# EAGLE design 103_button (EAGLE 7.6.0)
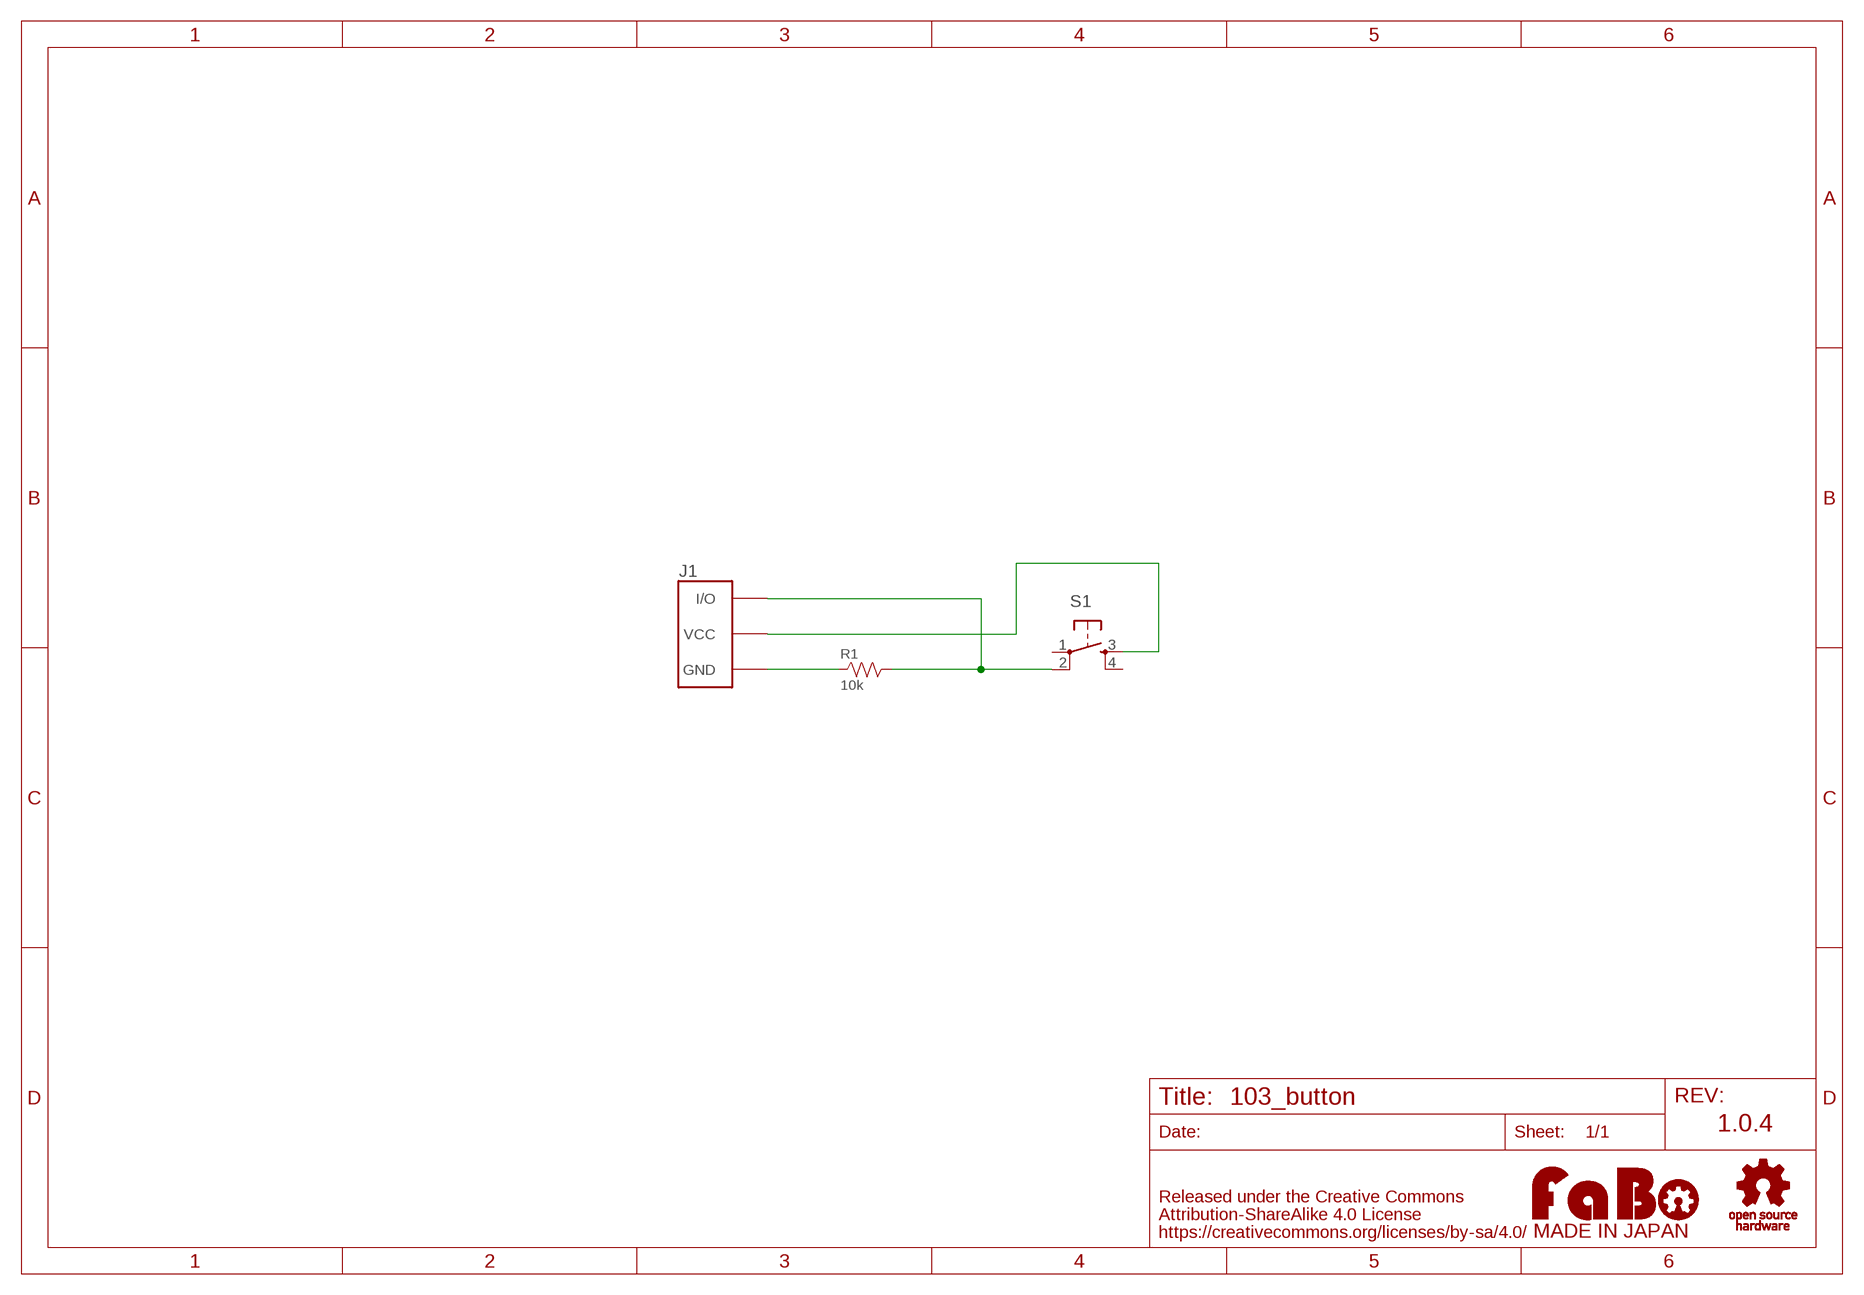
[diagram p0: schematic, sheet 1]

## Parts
J1  FABO_BRICK_3PIN  [FABO_BRICK_3PIN]
R1  10k  RESISTOR-AXL-REGULAR  [AXL-REGULAR]
S1  TACT-SWITCH-12MM  [1273HA-160G-G]
U$2  LOGO_OSHW-M_BOTTOM  [LOGO_OSHW_M_BOTTOM]
U$3  LOGO_FABO-M_BOTTOM  [LOGO_FABO_MS_BOTTOM]

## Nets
GND: J1.GND R1.1
N$1: J1.VCC S1.3
N$4: J1.I/O R1.2 S1.2
Unconnected: S1.1 S1.4

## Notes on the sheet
- 1.0.4

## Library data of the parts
J1 = FaBo-Template:FABO_BRICK_3PIN: FaBo Brick 3pin
R1 = FaBo-Resistors:RESISTOR: RESISTOR
S1 = FaBo-Switch:TACT-SWITCH
U$2 = FaBo-etc:LOGO_OSHW
U$3 = FaBo-etc:LOGO_FABO

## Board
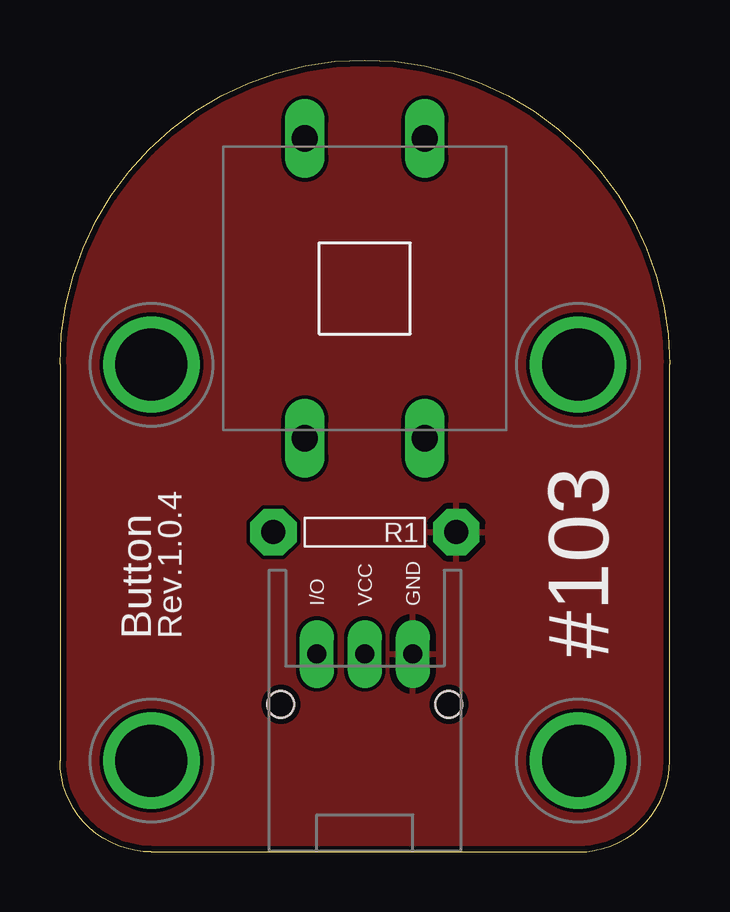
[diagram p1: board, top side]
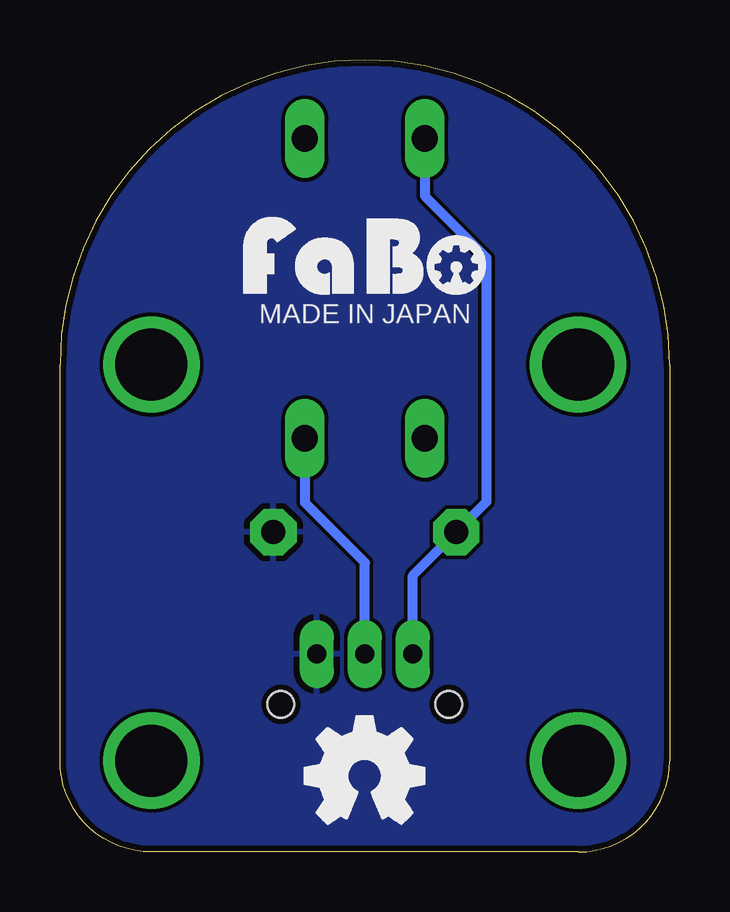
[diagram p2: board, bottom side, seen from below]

Size 25.4 x 33.02 mm. Coordinates in mm from the lower left corner, seen from the top.
Copper layers (1*16): Top 0.035mm / dielectric 1.5mm / Bottom 0.035mm
Design rules "SeeedStudio_2layer_DRU_no_angle_20140221": minimum track width 6mil, minimum drill 12mil, track to track 6mil, track to pad 6mil, pad to pad 6mil, via to via 6mil, smd to smd 0mil, copper to edge 10mil, drill to drill 10mil, minimum pad ring 10mil, minimum via ring 6mil, stop-mask expansion 2mil, vias tented up to drill 100mil, thermal gap 10mil

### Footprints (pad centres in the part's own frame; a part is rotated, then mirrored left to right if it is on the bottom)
FABO_BRICK_3PIN = drill 0.8 pad 1.422 long: GND 2,-8.255; I/O -2,-8.255; VCC 0,-8.255 | drill 3 pad 3.81: P$1 -8.89,3.81; P$2 8.89,3.81; P$3 -8.89,-12.7; P$4 8.89,-12.7 | hole 1.1: -3.5,-10.355; 3.5,-10.355
AXL-REGULAR = drill 1 pad 1.93 octagon: 1 -3.81,0; 2 3.81,0
1273HA-160G-G = drill 1.1 long: 1 -6.25,2.5; 2 6.25,2.5; 3 -6.25,-2.5; 4 6.25,-2.5

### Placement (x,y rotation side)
J1  12.7,16.51 0 top
R1  12.7,13.34 180 top
S1  12.7,23.5 90 top
U$2  12.7,3.17 0 top
U$3  12.7,22.86 0 top

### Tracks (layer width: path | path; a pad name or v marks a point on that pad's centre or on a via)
GND
  pour Bottom: 0,0 25.4,0 25.4,33.02 0,33.02
  pour Top: 0,0 25.4,0 25.4,33.02 0,33.02
N$1
  Bottom 0.406: J1.VCC 12.7,12.06 15.2,14.56 S1.3
N$4
  Bottom 0.406: J1.I/O 10.7,11.53 R1.2 7.62,14.61 7.62,24.77 10.2,27.34 S1.2

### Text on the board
tPlace: #103 | Button | Rev.1.0.4
bPlace: MADE IN JAPAN

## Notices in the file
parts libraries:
FaBo-etc: Released under the Creative Commons Attribution-ShareAlike 4.0 License
https://creativecommons.org/licenses/by-sa/4.0
FaBo-etc: Released under the Creative Commons
